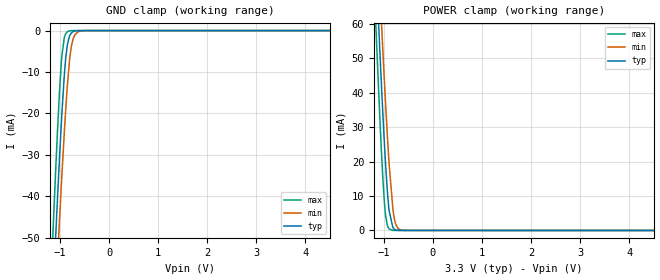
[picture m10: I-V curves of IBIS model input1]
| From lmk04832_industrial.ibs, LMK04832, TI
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|   input1 Model
[Model]   input1
Model_type   Input
Vinl = 0.4
Vinh = 1.2
|   typ   min   max
C_comp   0.3074pF   0.3004pF   0.3116pF
|  Where Nom  PVT is Nominal Process,   3.3V,  25C
|   Fast PVT is Strong Process,   3.45V, -40C
|   Slow PVT is Weak Process,   3.15V, 85C
[Model spec]
|subparameter
Vinl   0.400   0.370   0.430
Vinh   1.200   1.170   1.230
[Voltage Range]   3.3   3.15   3.45
|Junction Temperature
[Temperature Range]   25   85   -40
[Power Clamp Reference]   3.3   3.15   3.45
[GND Clamp Reference]   0   0   0
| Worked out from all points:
|   GND clamp passes 1 mA (typ) near -0.79 V on its own axis
|   POWER clamp passes 1 mA (typ) near -0.82 V on its own axis
[GND Clamp]
|   Voltage   I(typ)   I(min)   I(max)
-3.3V     -672.7mA   -647.6mA   -705.9mA
-1.171V   -70.78mA   -84.12mA   -55.94mA
-1.092V   -50.35mA   -64.75mA   -34.3mA
-1.053V   -40.5mA    -55.3mA    -24.2mA
-1.013V   -31.05mA   -46.07mA   -15.01mA
-963.6mV  -20.09mA   -34.97mA   -6.05mA
-914.1mV  -10.81mA   -24.59mA   -1.678mA
-884.4mV  -6.571mA   -18.87mA   -740.3uA
-815.1mV  -1.572mA   -8.086mA   -76.58uA
-726mV    -201.3uA   -1.759mA   -3.647uA
-547.8mV  -2.202uA   -43.96uA   -1.835uA
6.6V      0A         0A         0A
[POWER Clamp]
|   Voltage   I(typ)   I(min)   I(max)
-3.3V     834.6mA    808.2mA    869.6mA
-1.171V   80.82mA    97.59mA    62.56mA
-1.142V   71.19mA    88.42mA    52.41mA
-1.082V   52.45mA    70.41mA    33mA
-1.053V   43.43mA    61.62mA    24.01mA
-1.023V   34.75mA    53.02mA    15.86mA
-973.5mV  21.42mA    39.24mA    5.581mA
-894.3mV  5.863mA    19.63mA    449.1uA
-815.1mV  819.3uA    6.103mA    27.6uA
-785.4mV  360uA      3.397mA    17.28uA
-636.9mV  14.5uA     106.3uA    13.71uA
6.6V      0A         0A         0A
